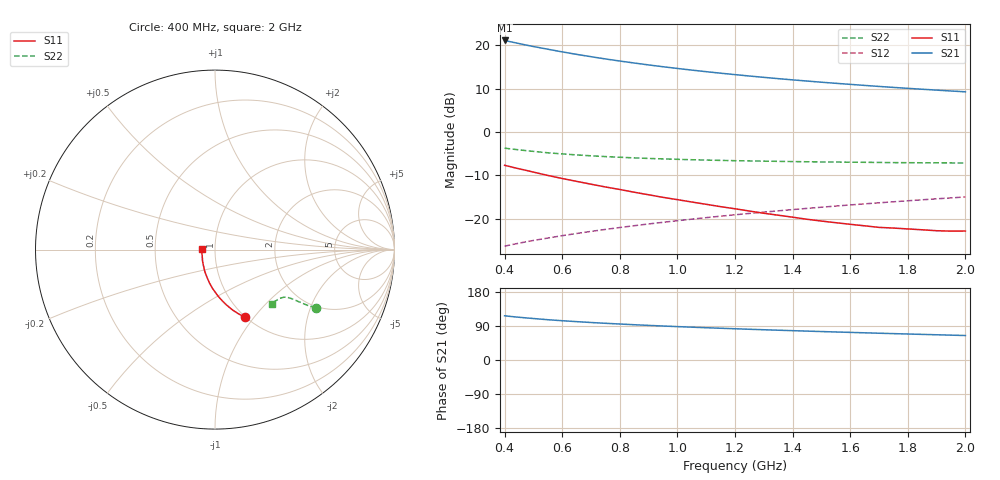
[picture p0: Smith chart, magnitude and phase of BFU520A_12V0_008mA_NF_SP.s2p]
! Filename:  P:\Prog\Test\Noise\ATS_data\Testdata_Net\06 Compressed Noise after Statistics\BFU520A_APG2013_30_A05_12p0V_008mA_NF_CM01_D.sf
! Date/Time: Wed 24/Apr/2013 20:06:21
! BFU520A_APG2013_30_A05_12p0V_1to20mA_NF_CM01_Bias5_R.sf
! Noise Parameter Data File
! BFU520A_APG2013_30_A05_12p0V_1to20mA_NF_CM01
! Date/time: Thu Apr 11 10:46:45 2013
! VAR V_out= 12.001000
! VAR I_out= 8.000000
! VAR V_in= 0.815900
! VAR I_in= 0.079400
! Device data file deembeded for feedlines and parallel
! Original file: \06 Compressed Noise after Statistics\BFU520A_APG2013_30_A05_12p0V_008mA_NF_CM01_R.sf
! Feed-files: PR017V01_150413_Feed1.s2p, PR017V01_150413_Feed2.s2p
! Parallel-file: PR017V01_150413_Par.s2p
# MHz S MA R 50
!  Freq-MHz  S11-mag  S11-arg  S21-mag  S21-arg  S12-mag  S12-arg  S22-mag  S22-arg
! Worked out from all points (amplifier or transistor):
!   37 points, 400 MHz to 2 GHz, reference 50 ohm
!   highest |S21| = 21.1 dB at 400 MHz (marker M1)
!   |S21| within 3 dB of that: start of sweep to 631.6 MHz
!   unconditionally stable (mu >= 1): 1.45 GHz to end of sweep
!   at 500 MHz: K = 0.75, MSG = 22.4 dB, |S12| = -25.1 dB
!   at 1.1 GHz: K = 0.97, MSG = 16.9 dB, |S12| = -19.8 dB
!   at 2 GHz: K = 1.01, MAG = 11.6 dB, |S12| = -15.0 dB
!   lowest NFmin = 0.80 dB at 420 MHz
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400  0.4112 -66.1  11.37 116.6  0.04795 67.1  0.6492 -29.9
420  0.3967 -68.0  10.99 115.0  0.04956 67.0  0.6369 -30.2
440  0.3819 -69.8  10.64 113.5  0.05114 67.0  0.6258 -30.5
460  0.3689 -71.3  10.29 112.1  0.0527 67.0  0.6153 -30.8
480  0.3564 -73.0  9.976 110.7  0.05425 67.0  0.6047 -31.0
500  0.3434 -74.6  9.673 109.4  0.0558 67.0  0.5958 -31.2
550  0.3143 -78.4  9.007 106.3  0.05951 67.1  0.5738 -31.5
600  0.2898 -81.7  8.387 103.7  0.06337 67.3  0.5571 -31.7
650  0.2686 -84.8  7.854 101.2  0.06718 67.5  0.5424 -32.0
700  0.249 -87.8  7.38 98.9  0.07102 67.8  0.5298 -32.2
750  0.2314 -90.7  6.955 96.9  0.07487 68.0  0.5189 -32.4
800  0.2163 -93.7  6.58 94.9  0.07874 68.2  0.5095 -32.6
850  0.2012 -96.6  6.24 93.1  0.08262 68.4  0.5012 -32.8
950  0.1756 -102.2  5.654 89.7  0.09043 68.7  0.4877 -33.3
1050  0.155 -107.7  5.168 86.6  0.09835 69.0  0.4772 -33.8
1150  0.1371 -114.0  4.761 83.8  0.1064 69.0  0.4688 -34.4
1200  0.1296 -116.8  4.583 82.5  0.1105 69.1  0.4654 -34.8
1350  0.1092 -126.5  4.119 78.6  0.1226 69.0  0.4571 -36.0
1500  0.09349 -137.9  3.747 75.1  0.1351 68.8  0.45 -37.4
1650  0.08236 -149.7  3.441 71.8  0.1477 68.4  0.4456 -39.1
1750  0.07761 -158.8  3.263 69.6  0.156 68.2  0.442 -40.2
2000  0.07171 179.2  2.902 64.6  0.1774 67.2  0.4373 -43.4
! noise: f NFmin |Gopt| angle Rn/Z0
400  0.8402  0.08779  5.95  0.1226
460  0.7975  0.07323  16.65  0.117
600  0.9093  0.1046  17.16  0.1402
800  0.867  0.04437  55.08  0.1089
1000  0.8893  0.04175  75.59  0.1063
1200  0.9139  0.0343  84.75  0.1092
1400  0.9473  0.04471  137.2  0.1026
1600  0.9483  0.05051  168.8  0.0967
1800  0.9232  0.08104  -171.3  0.0943
2000  0.9479  0.1052  -166.3  0.091
